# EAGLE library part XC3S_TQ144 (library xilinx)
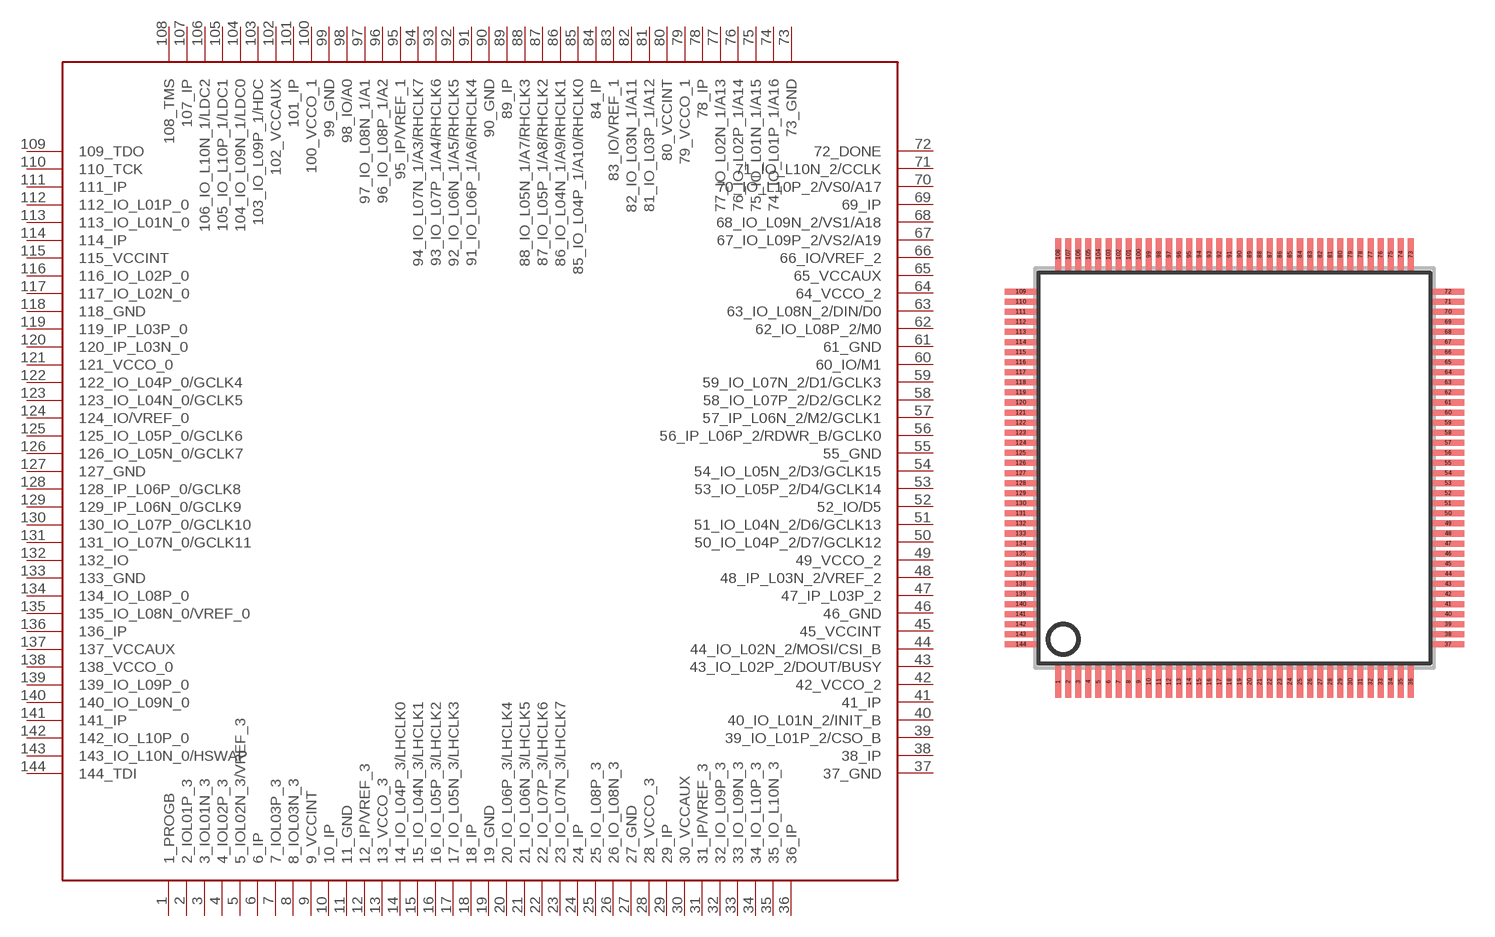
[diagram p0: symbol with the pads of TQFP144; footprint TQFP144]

Designator prefix -

## XC3S_TQ144  [TQFP144]
1  1_PROGB
2  2_IOL01P_3
3  3_IOL01N_3
4  4_IOL02P_3
5  5_IOL02N_3/VREF_3
6  6_IP
7  7_IOL03P_3
8  8_IOL03N_3
9  9_VCCINT
10  10_IP
11  11_GND
12  12_IP/VREF_3
13  13_VCCO_3
14  14_IO_L04P_3/LHCLK0
15  15_IO_L04N_3/LHCLK1
16  16_IO_L05P_3/LHCLK2
17  17_IO_L05N_3/LHCLK3
18  18_IP
19  19_GND
20  20_IO_L06P_3/LHCLK4
21  21_IO_L06N_3/LHCLK5
22  22_IO_L07P_3/LHCLK6
23  23_IO_L07N_3/LHCLK7
24  24_IP
25  25_IO_L08P_3
26  26_IO_L08N_3
27  27_GND
28  28_VCCO_3
29  29_IP
30  30_VCCAUX
31  31_IP/VREF_3
32  32_IO_L09P_3
33  33_IO_L09N_3
34  34_IO_L10P_3
35  35_IO_L10N_3
36  36_IP
37  37_GND
38  38_IP
39  39_IO_L01P_2/CSO_B
40  40_IO_L01N_2/INIT_B
41  41_IP
42  42_VCCO_2
43  43_IO_L02P_2/DOUT/BUSY
44  44_IO_L02N_2/MOSI/CSI_B
45  45_VCCINT
46  46_GND
47  47_IP_L03P_2
48  48_IP_L03N_2/VREF_2
49  49_VCCO_2
50  50_IO_L04P_2/D7/GCLK12
51  51_IO_L04N_2/D6/GCLK13
52  52_IO/D5
53  53_IO_L05P_2/D4/GCLK14
54  54_IO_L05N_2/D3/GCLK15
55  55_GND
56  56_IP_L06P_2/RDWR_B/GCLK0
57  57_IP_L06N_2/M2/GCLK1
58  58_IO_L07P_2/D2/GCLK2
59  59_IO_L07N_2/D1/GCLK3
60  60_IO/M1
61  61_GND
62  62_IO_L08P_2/M0
63  63_IO_L08N_2/DIN/D0
64  64_VCCO_2
65  65_VCCAUX
66  66_IO/VREF_2
67  67_IO_L09P_2/VS2/A19
68  68_IO_L09N_2/VS1/A18
69  69_IP
70  70_IO_L10P_2/VS0/A17
71  71_IO_L10N_2/CCLK
72  72_DONE
73  73_GND
74  74_IO_L01P_1/A16
75  75_IO_L01N_1/A15
76  76_IO_L02P_1/A14
77  77_IO_L02N_1/A13
78  78_IP
79  79_VCCO_1
80  80_VCCINT
81  81_IO_L03P_1/A12
82  82_IO_L03N_1/A11
83  83_IO/VREF_1
84  84_IP
85  85_IO_L04P_1/A10/RHCLK0
86  86_IO_L04N_1/A9/RHCLK1
87  87_IO_L05P_1/A8/RHCLK2
88  88_IO_L05N_1/A7/RHCLK3
89  89_IP
90  90_GND
91  91_IO_L06P_1/A6/RHCLK4
92  92_IO_L06N_1/A5/RHCLK5
93  93_IO_L07P_1/A4/RHCLK6
94  94_IO_L07N_1/A3/RHCLK7
95  95_IP/VREF_1
96  96_IO_L08P_1/A2
97  97_IO_L08N_1/A1
98  98_IO/A0
99  99_GND
100  100_VCCO_1
101  101_IP
102  102_VCCAUX
103  103_IO_L09P_1/HDC
104  104_IO_L09N_1/LDC0
105  105_IO_L10P_1/LDC1
106  106_IO_L10N_1/LDC2
107  107_IP
108  108_TMS
109  109_TDO
110  110_TCK
111  111_IP
112  112_IO_L01P_0
113  113_IO_L01N_0
114  114_IP
115  115_VCCINT
116  116_IO_L02P_0
117  117_IO_L02N_0
118  118_GND
119  119_IP_L03P_0
120  120_IP_L03N_0
121  121_VCCO_0
122  122_IO_L04P_0/GCLK4
123  123_IO_L04N_0/GCLK5
124  124_IO/VREF_0
125  125_IO_L05P_0/GCLK6
126  126_IO_L05N_0/GCLK7
127  127_GND
128  128_IP_L06P_0/GCLK8
129  129_IP_L06N_0/GCLK9
130  130_IO_L07P_0/GCLK10
131  131_IO_L07N_0/GCLK11
132  132_IO
133  133_GND
134  134_IO_L08P_0
135  135_IO_L08N_0/VREF_0
136  136_IP
137  137_VCCAUX
138  138_VCCO_0
139  139_IO_L09P_0
140  140_IO_L09N_0
141  141_IP
142  142_IO_L10P_0
143  143_IO_L10N_0/HSWAP
144  144_TDI

## Footprint TQFP144 (pad centres in mm)
QFP144 shrink quad flat pack, square (smd-ipc)
smd 0.3 x 1.6: 1 -8.75,-10.6; 2 -8.25,-10.6; 3 -7.75,-10.6; 4 -7.25,-10.6; 5 -6.75,-10.6; 6 -6.25,-10.6; 7 -5.75,-10.6; 8 -5.25,-10.6; 9 -4.75,-10.6; 10 -4.25,-10.6; 11 -3.75,-10.6; 12 -3.25,-10.6; 13 -2.75,-10.6; 14 -2.25,-10.6; 15 -1.75,-10.6; 16 -1.25,-10.6; 17 -0.75,-10.6; 18 -0.25,-10.6; 19 0.25,-10.6; 20 0.75,-10.6; 21 1.25,-10.6; 22 1.75,-10.6; 23 2.25,-10.6; 24 2.75,-10.6; 25 3.25,-10.6; 26 3.75,-10.6; 27 4.25,-10.6; 28 4.75,-10.6; 29 5.25,-10.6; 30 5.75,-10.6; 31 6.25,-10.6; 32 6.75,-10.6; 33 7.25,-10.6; 34 7.75,-10.6; 35 8.25,-10.6; 36 8.75,-10.6; 73 8.75,10.6; 74 8.25,10.6; 75 7.75,10.6; 76 7.25,10.6; 77 6.75,10.6; 78 6.25,10.6; 79 5.75,10.6; 80 5.25,10.6; 81 4.75,10.6; 82 4.25,10.6; 83 3.75,10.6; 84 3.25,10.6; 85 2.75,10.6; 86 2.25,10.6; 87 1.75,10.6; 88 1.25,10.6; 89 0.75,10.6; 90 0.25,10.6; 91 -0.25,10.6; 92 -0.75,10.6; 93 -1.25,10.6; 94 -1.75,10.6; 95 -2.25,10.6; 96 -2.75,10.6; 97 -3.25,10.6; 98 -3.75,10.6; 99 -4.25,10.6; 100 -4.75,10.6; 101 -5.25,10.6; 102 -5.75,10.6; 103 -6.25,10.6; 104 -6.75,10.6; 105 -7.25,10.6; 106 -7.75,10.6; 107 -8.25,10.6; 108 -8.75,10.6
smd 1.6 x 0.3: 37 10.6,-8.75; 38 10.6,-8.25; 39 10.6,-7.75; 40 10.6,-7.25; 41 10.6,-6.75; 42 10.6,-6.25; 43 10.6,-5.75; 44 10.6,-5.25; 45 10.6,-4.75; 46 10.6,-4.25; 47 10.6,-3.75; 48 10.6,-3.25; 49 10.6,-2.75; 50 10.6,-2.25; 51 10.6,-1.75; 52 10.6,-1.25; 53 10.6,-0.75; 54 10.6,-0.25; 55 10.6,0.25; 56 10.6,0.75; 57 10.6,1.25; 58 10.6,1.75; 59 10.6,2.25; 60 10.6,2.75; 61 10.6,3.25; 62 10.6,3.75; 63 10.6,4.25; 64 10.6,4.75; 65 10.6,5.25; 66 10.6,5.75; 67 10.6,6.25; 68 10.6,6.75; 69 10.6,7.25; 70 10.6,7.75; 71 10.6,8.25; 72 10.6,8.75; 109 -10.6,8.75; 110 -10.6,8.25; 111 -10.6,7.75; 112 -10.6,7.25; 113 -10.6,6.75; 114 -10.6,6.25; 115 -10.6,5.75; 116 -10.6,5.25; 117 -10.6,4.75; 118 -10.6,4.25; 119 -10.6,3.75; 120 -10.6,3.25; 121 -10.6,2.75; 122 -10.6,2.25; 123 -10.6,1.75; 124 -10.6,1.25; 125 -10.6,0.75; 126 -10.6,0.25; 127 -10.6,-0.25; 128 -10.6,-0.75; 129 -10.6,-1.25; 130 -10.6,-1.75; 131 -10.6,-2.25; 132 -10.6,-2.75; 133 -10.6,-3.25; 134 -10.6,-3.75; 135 -10.6,-4.25; 136 -10.6,-4.75; 137 -10.6,-5.25; 138 -10.6,-5.75; 139 -10.6,-6.25; 140 -10.6,-6.75; 141 -10.6,-7.25; 142 -10.6,-7.75; 143 -10.6,-8.25; 144 -10.6,-8.75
